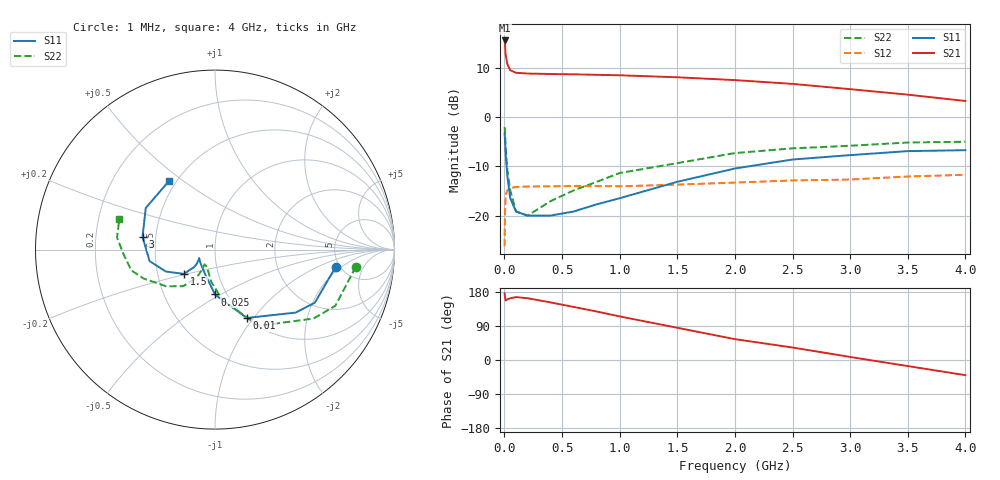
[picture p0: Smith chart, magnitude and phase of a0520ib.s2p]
!  MSA-0520 S PARAMETERS
!  Id=165mA  LAST UPDATED 07-22-92
# ghz s ma r 50
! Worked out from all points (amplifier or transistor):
!   18 points, 1 MHz to 4 GHz, reference 50 ohm
!   highest |S21| = 15.5 dB at 1 MHz (marker M1)
!   |S21| within 3 dB of that: start of sweep to 10.62 MHz
!   unconditionally stable (mu >= 1): 33.5 MHz to 1.48 GHz
!   at 10 MHz: K = 0.66, MSG = 14.2 dB, |S12| = -15.8 dB
!   at 600 MHz: K = 1.14, MAG = 9.0 dB, |S12| = -14.0 dB
!   at 4 GHz: K = 0.65, MSG = 7.5 dB, |S12| = -11.7 dB
!   S11 on the Smith chart (normalised r, x): 1 MHz: 4.65, -1.64; 10 MHz: 1.00, -0.93; 25 MHz: 0.88, -0.47; 1.5 GHz: 0.68, -0.19; 3 GHz: 0.42, +0.07; 4 GHz: 0.46, +0.44
0.001  0.68 -8.0  5.95 176.0  0.049 25.0  0.79 -7.0
0.003  0.63 -28.0  5.65 168.0  0.085 41.0  0.74 -25.0
0.005  0.57 -38.0  5.25 165.0  0.107 38.0  0.67 -35.0
0.01  0.42 -65.0  4.25 157.0  0.162 29.0  0.49 -60.0
0.025  0.25 -90.0  3.42 160.0  0.18 17.0  0.29 -81.0
0.05  0.15 -111.0  2.97 163.0  0.19 9.0  0.18 -97.0
0.1  0.11 -138.0  2.8 166.0  0.195 3.0  0.11 -113.0
0.2  0.1 -152.0  2.75 163.0  0.197 1.0  0.1 -125.0
0.4  0.1 -152.0  2.72 152.0  0.198 -2.0  0.14 -123.0
0.6  0.11 -147.0  2.7 140.0  0.199 -4.0  0.18 -123.0
0.8  0.13 -142.0  2.67 128.0  0.199 -6.0  0.22 -127.0
1  0.15 -140.0  2.64 115.0  0.198 -8.0  0.27 -131.0
1.5  0.22 -142.0  2.52 85.0  0.206 -12.0  0.34 -143.0
2  0.3 -156.0  2.36 55.0  0.216 -16.0  0.43 -158.0
2.5  0.37 -170.0  2.16 33.0  0.227 -18.0  0.48 -166.0
3  0.41 170.0  1.91 8.0  0.232 -23.0  0.51 -177.0
3.5  0.45 149.0  1.68 -16.0  0.249 -31.0  0.55 173.0
4  0.46 124.0  1.45 -40.0  0.259 -39.0  0.56 162.0
